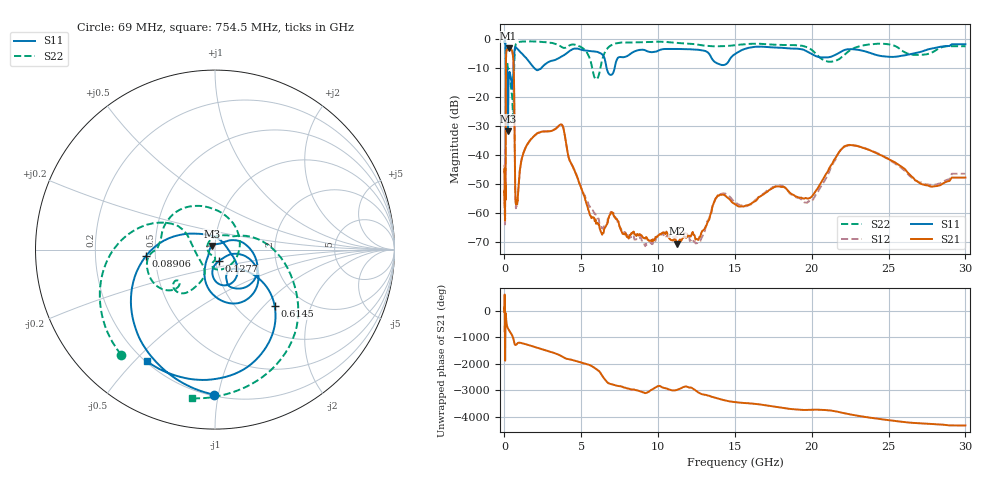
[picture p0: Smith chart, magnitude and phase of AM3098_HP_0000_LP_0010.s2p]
! Date/Time: Thu, Feb 28, 2019 8:30 AM
! Network Analyzer: Agilent Technologies E8364B Rev: A.07.50.67
! Sweep from 0.010 to 30.000 GHz, 1601 Points, Sweep Type: LOG
! Power Supply: 5.022 V, 0.002 A
# Hz S DB R 50
!freq MagS11 AngS11 MagS21 AngS21 MagS12 AngS12 MagS22 AngS22
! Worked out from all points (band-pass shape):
!   1601 points, 10 MHz to 30 GHz, reference 50 ohm
!   highest |S21| = -3.01 dB at 266.5 MHz (marker M1); lowest = -70.4 dB at 11.25 GHz (marker M2)
!   |S21| within 3 dB of the highest: 103.6 MHz to 562.6 MHz (459 MHz wide, 138 % of centre)
!   lowest |S11| = -31.7 dB at 227 MHz (marker M3), VSWR 1.05, Z = 48.3 + j1.96 ohm
!   |S11| at or under -10 dB: 175.6 MHz to 587.7 MHz (412.2 MHz wide, 108 % of centre); 1.966 GHz to 2.38 GHz (414.1 MHz wide, 19.1 % of centre); 6.653 GHz to 7.164 GHz (511.2 MHz wide, 7.4 % of centre)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
!   |S22| runs from -28.9 to -0.5 dB; largest |S21 - S12| = 0.011
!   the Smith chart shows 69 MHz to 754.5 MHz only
!   S11 on the Smith chart (normalised r, x): 69 MHz: 0.21, -0.97; 89.06 MHz: 0.44, -0.04; 127.7 MHz: 1.03, -0.13; 614.5 MHz: 1.45, -1.16; 754.5 MHz: 0.21, -0.54
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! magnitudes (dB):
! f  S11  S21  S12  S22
! 10 MHz  -0.3  -45.9  -44.0  -0.5
! 38.04 MHz  -0.5  -61.6  -63.5  -0.8
! 69 MHz  -1.9  -52.3  -50.6  -2.1
! 89.06 MHz  -8.2  -18.2  -18.2  -10.0
! 97.94 MHz  -24.4  -7.8  -7.8  -17.8
! 127.7 MHz  -23.4  -4.0  -3.9  -11.2
! 144.7 MHz  -13.2  -3.6  -3.5  -10.1
! 187.7 MHz  -11.7  -3.4  -3.4  -8.3
! 227 MHz  -31.7  -3.1  -3.1  -9.8
! 266.5 MHz  -14.8  -3.0  -3.0  -10.2
! 550.5 MHz  -14.9  -5.4  -5.4  -25.1
! 614.5 MHz  -6.8  -12.6  -12.5  -14.4
! 699.9 MHz  -2.7  -51.6  -52.9  -2.5
! 754.5 MHz  -2.8  -56.7  -58.2  -1.5
! 2.084 GHz  -10.5  -32.6  -32.6  -0.7
! 3.723 GHz  -5.9  -29.4  -29.4  -2.6
! 5.989 GHz  -4.2  -63.6  -61.2  -13.7
! 7.926 GHz  -5.9  -67.6  -67.3  -1.0
! 11.25 GHz  -3.3  -70.4  -68.1  -1.2
! 19.8 GHz  -4.5  -54.9  -55.7  -3.0
! 22.67 GHz  -3.4  -36.5  -36.6  -3.2
! 30 GHz  -1.6  -47.7  -46.4  -2.3
